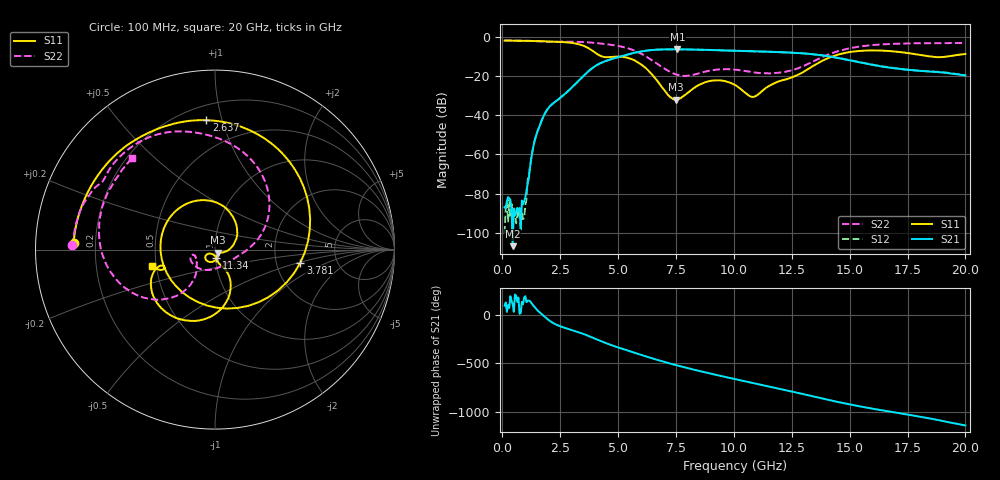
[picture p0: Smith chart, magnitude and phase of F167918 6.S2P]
!  2-Port S-parameters saved by WinCal
! VAR MeasName=S-Parameters (CALIBRATED_DATA) read from VNA (N5242A)
! VAR MeasDate=2016-11-22 10:25:08
! VAR NAME=F167918 6
! VAR FILENAME=F167918 6.S2P
! VAR DATE=2016-11-22 10:25:08
! VAR PHYS_PORTS=1,2
# Hz S DB R 50
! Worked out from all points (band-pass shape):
!   401 points, 100 MHz to 20 GHz, reference 50 ohm
!   highest |S21| = -6.49 dB at 7.562 GHz (marker M1); lowest = -106.7 dB at 448.2 MHz (marker M2)
!   |S21| within 3 dB of the highest: 5.303 GHz to 13.75 GHz (8.448 GHz wide, 88.7 % of centre)
!   lowest |S11| = -32.2 dB at 7.513 GHz (marker M3), VSWR 1.05, Z = 51.8 - j1.75 ohm
!   |S11| at or under -10 dB: 4.269 GHz to 14.29 GHz (10.02 GHz wide, 108 % of centre); 18.39 GHz to 19.3 GHz (902.9 MHz wide, 4.79 % of centre)
!   |S22| runs from -20.1 to -2.0 dB; largest |S21 - S12| = 0.0049
!   S11 on the Smith chart (normalised r, x): 100 MHz: 0.12, +0.02; 2.637 GHz: 0.30, +0.89; 3.781 GHz: 2.74, -0.52; 11.34 GHz: 1.01, -0.09; 20 GHz: 0.48, -0.10
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1e8  -2.07 177.3  -86.86 91.4  -100.08 62.2  -2.00 178.3
4.4825e8  -2.11 168.0  -106.69 105.5  -90.15 -106.3  -2.05 172.6
9.4575e8  -2.19 154.6  -83.72 177.4  -92.64 -109.4  -2.13 164.5
1.3935e9  -2.28 141.6  -53.11 77.4  -53.05 75.9  -2.33 157.1
1.64225e9  -2.34 133.7  -44.40 15.7  -44.44 14.7  -2.46 153.0
2.63725e9  -2.82 93.8  -29.90 -132.8  -29.91 -133.2  -2.60 138.5
3.43325e9  -4.38 34.8  -20.85 165.7  -20.88 165.6  -2.77 121.4
3.7815e9  -6.36 -8.8  -17.07 133.5  -17.06 133.5  -3.01 112.6
4.1795e9  -9.50 -78.7  -13.93 93.4  -13.87 93.3  -3.47 102.1
4.677e9  -10.42 -169.7  -11.64 47.3  -11.59 47.0  -4.18 87.6
5.672e9  -11.94 83.0  -8.36 -30.9  -8.39 -31.3  -6.99 49.2
6.7665e9  -23.70 -7.2  -6.63 -113.0  -6.65 -113.1  -14.50 1.9
7.51275e9  -32.20 -43.4  -6.50 -162.4  -6.51 -162.4  -19.31 -34.9
7.5625e9  -32.06 -44.1  -6.49 -165.5  -6.51 -165.5  -19.51 -38.1
8.856e9  -22.90 -105.1  -6.81 118.4  -6.80 118.4  -17.63 -122.8
1.005e10  -24.69 -148.1  -7.24 54.2  -7.25 54.3  -16.86 -161.9
1.079625e10  -30.74 -117.3  -7.51 15.4  -7.50 15.6  -18.08 -166.9
1.13435e10  -26.62 -81.1  -7.68 -13.0  -7.69 -12.8  -18.67 -160.5
1.338325e10  -15.26 -62.2  -8.96 -122.0  -8.94 -121.5  -12.91 -125.0
1.5025e10  -7.85 -102.7  -12.19 152.4  -12.06 152.7  -5.91 -150.1
1.67165e10  -7.40 -144.6  -15.79 80.1  -15.73 79.8  -3.82 175.9
2e10  -8.86 -165.5  -19.80 -63.5  -19.66 -64.0  -3.26 132.2
